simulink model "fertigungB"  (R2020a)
settings: Solver=FixedStepDiscrete  StartTime=0.0  StopTime=25.1  RelTol=1e-3  EnableMultiTasking=on

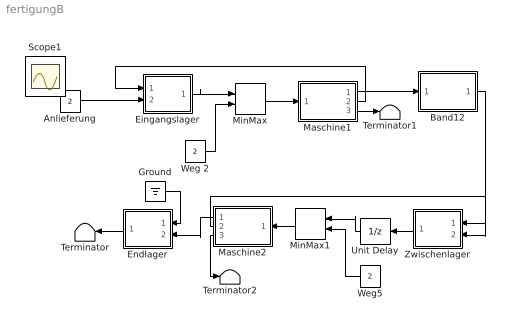
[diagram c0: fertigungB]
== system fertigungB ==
  Anlieferung : Constant  Value=2
  Band12 : Subsystem  mask{ndelay=3, dt=1, t0=0.1}
      mask prompts: ndelay "Transit time"; dt "Sample Period"; t0 "Start Time"
  Eingangslager : Subsystem  mask{m0=7, dt=1, t0=0.1}
      mask prompts: m0 "Initial Value"; dt "Sample Period"; t0 "Start Time"
  Endlager : Subsystem  mask{m0=0, dt=1, t0=0.1}
      mask prompts: m0 "Initial Value"; dt "Sample Period"; t0 "Start Time"
  Ground : Ground
  Maschine1 : Subsystem  mask(Oven){cookingtime=2, capacity=4, initload=0, dt=1, t0=0.1}
      mask prompts: cookingtime "Cooking time"; initload "Initial load"; dt "Sample Period"; t0 "Start Time"
  Maschine2 : Subsystem  mask(Oven){cookingtime=1, capacity=2, initload=0, dt=1, t0=0.1}
      mask prompts: cookingtime "Cooking time"; initload "Initial load"; dt "Sample Period"; t0 "Start Time"
  MinMax : MinMax  Inputs=2  InputSameDT=on  SaturateOnIntegerOverflow=on
  MinMax1 : MinMax  Inputs=2  InputSameDT=on  SaturateOnIntegerOverflow=on
  Terminator : Terminator
  Terminator1 : Terminator
  Terminator2 : Terminator
  Unit Delay : UnitDelay  SampleTime=-1  HasFrameUpgradeWarning=on
  Weg 2 : Constant  Value=2
  Weg5 : Constant  Value=2
  Zwischenlager : Subsystem  mask{m0=0, dt=1, t0=0.1}
      mask prompts: m0 "Initial Value"; dt "Sample Period"; t0 "Start Time"
  Scope1 : Scope
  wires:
  Anlieferung/1 -> Eingangslager/2(In2)
  MinMax/1 -> Maschine1/1(in)
  Eingangslager/1(Out1) -> MinMax/1
  Weg 2/1 -> MinMax/2
  Maschine1/1(out) -> Band12/1(In)
  MinMax1/1 -> Maschine2/1(in)
  Weg5/1 -> MinMax1/2
  Maschine2/1(out) -> Endlager/2(In2)
  Maschine1/2(increment) -> Eingangslager/1(In1)
  Endlager/1(Out1) -> Terminator/1
  Maschine1/3(load) -> Terminator1/1
  Zwischenlager/1(Out1) -> Unit Delay/1
  Band12/1(Out) -> Zwischenlager/2(In2)
  Maschine2/2(increment) -> Zwischenlager/1(In1)
  Unit Delay/1 -> MinMax1/1
  Maschine2/3(load) -> Terminator2/1
  Ground/1 -> Endlager/1(In1)

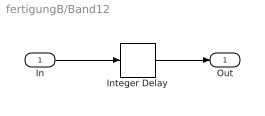
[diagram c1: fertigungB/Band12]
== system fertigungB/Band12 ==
  In : Inport
  Integer Delay : Delay  DelayLength=ndelay  SampleTime=[dt,t0]
  Out : Outport
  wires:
  Integer Delay/1 -> Out/1
  In/1 -> Integer Delay/1

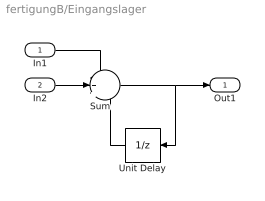
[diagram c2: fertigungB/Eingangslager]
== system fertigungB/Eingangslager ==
  In1 : Inport
  In2 : Inport  Port=2
  Sum : Sum  Inputs=-++  SaturateOnIntegerOverflow=on
  Unit Delay : UnitDelay  InitialCondition=m0  SampleTime=[dt, t0]  HasFrameUpgradeWarning=on
  Out1 : Outport
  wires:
  Unit Delay/1 -> Sum/3
  In2/1 -> Sum/2
  Sum/1 -> Unit Delay/1, Out1/1
  In1/1 -> Sum/1

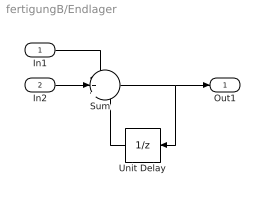
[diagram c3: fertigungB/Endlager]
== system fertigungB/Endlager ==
  In1 : Inport
  In2 : Inport  Port=2
  Sum : Sum  Inputs=-++  SaturateOnIntegerOverflow=on
  Unit Delay : UnitDelay  InitialCondition=m0  SampleTime=[dt, t0]  HasFrameUpgradeWarning=on
  Out1 : Outport
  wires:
  Unit Delay/1 -> Sum/3
  In2/1 -> Sum/2
  Sum/1 -> Unit Delay/1, Out1/1
  In1/1 -> Sum/1

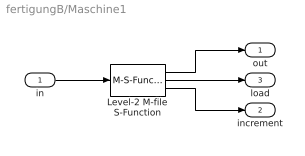
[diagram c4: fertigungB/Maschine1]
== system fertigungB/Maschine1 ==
  in : Inport
  Level-2 M-file S-Function : M-S-Function  FunctionName=sfun_oven  Parameters=capacity, cookingtime, initload, dt, t0
  out : Outport
  increment : Outport  Port=2
  load : Outport  Port=3
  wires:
  Level-2 M-file S-Function/3 -> increment/1
  Level-2 M-file S-Function/2 -> load/1
  Level-2 M-file S-Function/1 -> out/1
  in/1 -> Level-2 M-file S-Function/1

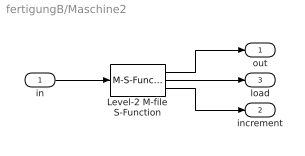
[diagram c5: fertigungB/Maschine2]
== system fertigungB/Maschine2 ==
  in : Inport
  Level-2 M-file S-Function : M-S-Function  FunctionName=sfun_oven  Parameters=capacity, cookingtime, initload, dt, t0
  out : Outport
  increment : Outport  Port=2
  load : Outport  Port=3
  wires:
  Level-2 M-file S-Function/3 -> increment/1
  Level-2 M-file S-Function/2 -> load/1
  Level-2 M-file S-Function/1 -> out/1
  in/1 -> Level-2 M-file S-Function/1

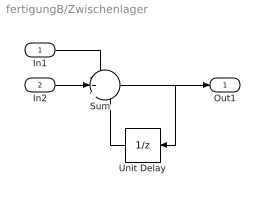
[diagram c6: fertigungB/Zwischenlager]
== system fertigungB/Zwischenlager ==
  In1 : Inport
  In2 : Inport  Port=2
  Sum : Sum  Inputs=-++  SaturateOnIntegerOverflow=on
  Unit Delay : UnitDelay  InitialCondition=m0  SampleTime=[dt, t0]  HasFrameUpgradeWarning=on
  Out1 : Outport
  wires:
  Unit Delay/1 -> Sum/3
  In2/1 -> Sum/2
  Sum/1 -> Unit Delay/1, Out1/1
  In1/1 -> Sum/1
